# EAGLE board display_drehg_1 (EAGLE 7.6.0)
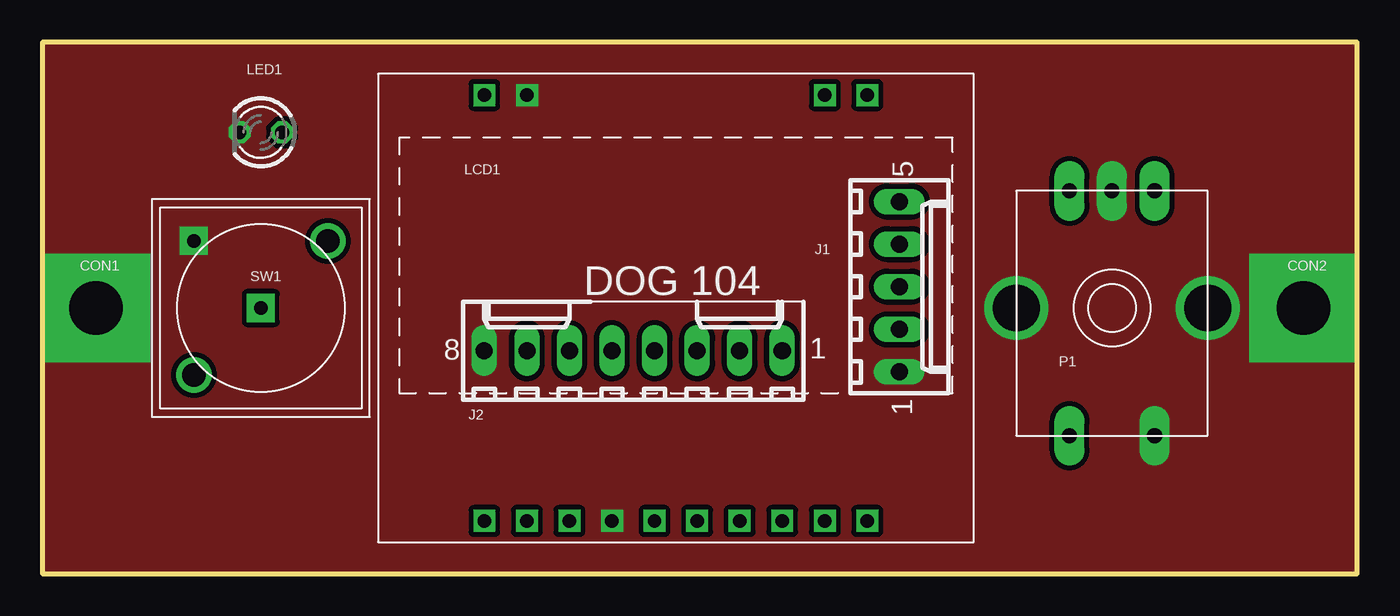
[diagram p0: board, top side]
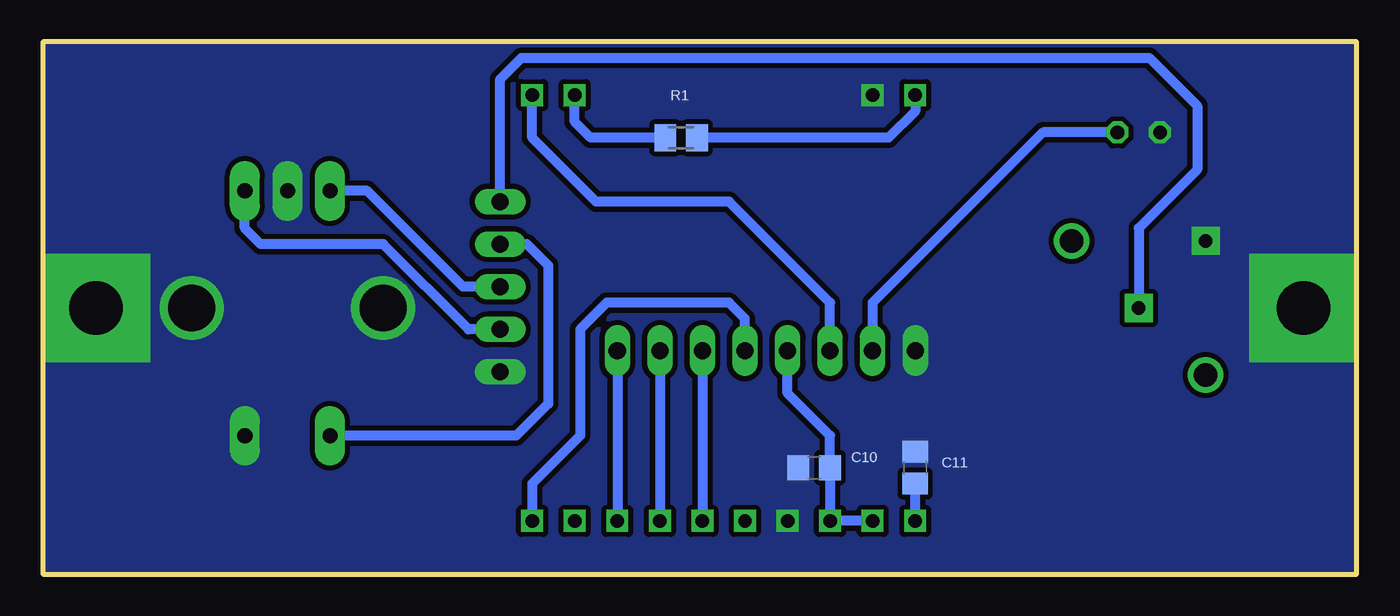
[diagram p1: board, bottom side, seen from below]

Size 78.42 x 31.75 mm. Coordinates in mm from the lower left corner, seen from the top.
Outline: 0,31.75 78.42,31.75 78.42,0 0,0 0,31.75
Copper layers (1*16): Top 0.035mm / dielectric 1.5mm / Bottom 0.035mm
Design rules "default *": minimum track width 10mil, minimum drill 24mil, track to track 8mil, track to pad 8mil, pad to pad 8mil, via to via 8mil, smd to smd 8mil, copper to edge 0mil, drill to drill 8mil, minimum pad ring 10mil, minimum via ring 8mil, stop-mask expansion 4mil, vias tented up to drill 0mil, thermal gap 10mil

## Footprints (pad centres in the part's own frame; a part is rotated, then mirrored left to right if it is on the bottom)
C0805 = smd 1.3 x 1.5: 1 -0.95,0; 2 0.95,0
HOLE3 = drill 3.2 pad 6.452 square: 1 0,0
6410-05 = drill 1.016 long: 1 5.08,0; 2 2.54,0; 3 0,0; 4 -2.54,0; 5 -5.08,0
6410-08 = drill 1.016 long: 1 8.89,0; 2 6.35,0; 3 3.81,0; 4 1.27,0; 5 -1.27,0; 6 -3.81,0; 7 -6.35,0; 8 -8.89,0
LCD_DOG_104 = drill 0.8 square: 1 0,0; 2 2.54,0; 9 20.32,0; 10 22.86,0; 11 22.86,25.4; 12 20.32,25.4; 13 17.78,25.4; 14 15.24,25.4; 15 12.7,25.4; 16 10.16,25.4; 17 7.62,25.4; 18 5.08,25.4; 19 2.54,25.4; 20 0,25.4
LED3MM = drill 0.813 octagon: A -1.27,0; K 1.27,0
DREHG = drill 0.9 pad 1.778 long: 1 3.175,14.605; 2 5.715,14.605; 3 8.255,14.605; 4 3.175,0; 5 8.255,0 | drill 2.8: 6 0,7.62 | drill 2.8 pad 3.81: 7 11.43,7.62
M0805 = smd 1.3 x 1.6: 1 -0.95,0; 2 0.95,0
MTG = drill 0.8 pad 1.676 square: 1 0,0; 2 -4,4 | drill 1.4: P$3 -4,-4; P$4 4,4

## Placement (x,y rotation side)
C10  1u  [C0805]  32.38,6.35 0 bottom
C11  1u  [C0805]  26.35,6.35 270 bottom
CON1  [HOLE3]  3.17,15.88 0 top
CON2  [HOLE3]  75.25,15.88 0 top
J1  Dreh  [6410-05]  51.12,17.14 270 top
J2  LCD  [6410-08]  35.24,13.34 0 top
LCD1  LCDDOG104NSPI  [LCD_DOG_104]  49.21,28.57 180 top
LED1  TX  [LED3MM]  13.02,26.35 180 top
P1  DREHGEBER  [DREHG]  58.1,8.26 0 top
R1  33  [M0805]  40.32,26.04 0 bottom
SW1  [MTG]  13.02,15.88 0 top

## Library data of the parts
C10 C11 = rcl; R: X5R-G0603 1,0/25
CON1 CON2 P1 SW1 = lindenau
J1 J2 = con-molex; OC_FARNELL: unknown; OC_NEWARK: unknown
LCD1 = lindenau; R: EA DOGS104W-A; R1: EA LED36X28-A; R2: SPL 20
LED1 = led
R1 = rcl

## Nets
5V: J2.6 LCD1.1
GND: C10.1 C11.1 CON1.1 CON2.1 J1.1 J2.8 LCD1.9 LCD1.14 LED1.K P1.2 P1.5 P1.6 P1.7 SW1.2
N$1: LCD1.2 R1.1
N$2: J1.5 SW1.1
N$3: J1.3 P1.1
N$4: LCD1.10 R1.2
N$5: J1.2 P1.3
N$6: J1.4 P1.4
N$7: J2.7 LED1.A
N$11: C11.2 LCD1.11
RC4: J2.3 LCD1.16
RC5: J2.2 LCD1.17
RC6: J2.1 LCD1.18
RC7: J2.4 LCD1.20
VDD: C10.2 J2.5 LCD1.12 LCD1.13

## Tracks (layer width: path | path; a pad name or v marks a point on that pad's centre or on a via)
5V
  Bottom 0.61: J2.6 31.43,16.19 37.47,22.23 45.4,22.23 49.21,26.04 LCD1.1
GND
  pour Top (isolate 0.305, no thermals): 0,31.75 78.42,31.75 78.42,0 0,0
  pour Bottom (isolate 0.305, no thermals): 0,31.75 78.42,31.75 78.42,0 0,0
N$1
  Bottom 0.61: R1.1 45.72,26.04 46.67,26.99 LCD1.2
N$2
  Bottom 0.61: J1.5 51.12,29.53 49.85,30.8 12.38,30.8 9.53,27.94 9.53,24.13 13.02,20.64 SW1.1
N$3
  Bottom 0.61: J1.3 53.34,17.14 59.05,22.86 P1.1
N$4
  Bottom 0.61: LCD1.10 26.35,27.62 27.94,26.04 R1.2
N$5
  Bottom 0.61: J1.2 53.02,14.61 58.1,19.68 65.41,19.68 66.36,20.64 P1.3
N$6
  Bottom 0.61: J1.4 49.53,19.68 48.26,18.41 48.26,10.16 50.16,8.26 P1.4
N$7
  Bottom 0.61: LED1.A 18.73,26.35 28.89,16.19 J2.7
N$11
  Bottom 0.61: LCD1.11 C11.2
RC4
  Bottom 0.61: J2.3 LCD1.16
RC5
  Bottom 0.61: J2.2 LCD1.17
RC6
  Bottom 0.61: J2.1 LCD1.18
RC7
  Bottom 0.61: J2.4 36.51,15.24 37.47,16.19 44.77,16.19 46.35,14.61 46.35,8.26 49.21,5.4 LCD1.20
VDD
  Bottom 0.61: LCD1.12 LCD1.13 C10.2 31.43,8.26 33.97,10.79 J2.5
